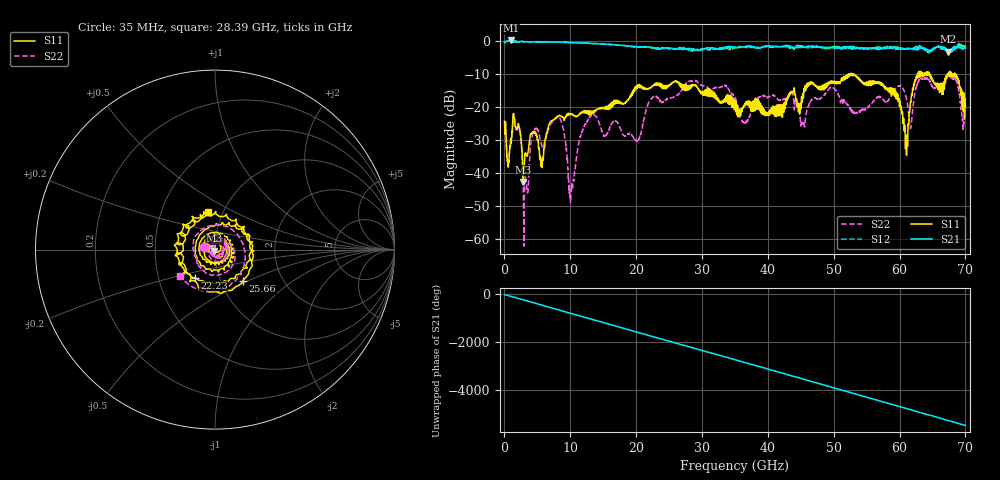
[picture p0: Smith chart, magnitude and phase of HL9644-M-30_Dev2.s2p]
! 7/2/2021 9:55:46 AM
! H:\PRODUCTION_DATA\TEMP_S2P.S2P
! CHANNEL.1
! TR.MEASUREMENT
! CORRECTED.DATA
# GHZ S RI R 50.0
! FREQ.GHZ  S11RE  S11IM  S21RE  S21IM  S12RE  S12IM  S22RE  S22IM
!; PortSelection: Port_12
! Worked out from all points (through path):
!   2000 points, 35 MHz to 70 GHz, reference 50 ohm
!   highest |S21| = 0.04 dB at 1.015 GHz (marker M1); lowest = -3.4 dB at 67.34 GHz (marker M2)
!   group delay of S21, straight-line fit = 217 ps
!   lowest |S11| = -42.8 dB at 2.87 GHz (marker M3), VSWR 1.01, Z = 49.6 - j0.614 ohm
!   |S11| at or under -10 dB: start of sweep to 52.53 GHz; 52.72 GHz to 62.72 GHz (9.998 GHz wide, 17.3 % of centre); 64.56 GHz to 67.42 GHz (2.861 GHz wide, 4.34 % of centre)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
!   |S22| runs from -62.3 to -10.4 dB; largest |S21 - S12| = 0.14
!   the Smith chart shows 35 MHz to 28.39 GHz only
!   S11 on the Smith chart (normalised r, x): 35 MHz: 0.89, +0.03; 22.23 GHz: 0.76, -0.25; 25.66 GHz: 1.27, -0.47; 28.39 GHz: 0.85, +0.37
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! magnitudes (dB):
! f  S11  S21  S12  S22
! 35 MHz  -24.5  -0.6  -0.6  -24.4
! 1.015 GHz  -29.6  0.0  -0.1  -29.6
! 2.205 GHz  -26.3  -0.4  -0.5  -26.7
! 2.87 GHz  -42.8  -0.3  -0.3  -45.0
! 3.29 GHz  -34.1  -0.3  -0.3  -42.1
! 4.515 GHz  -27.5  -0.4  -0.4  -27.2
! 5.705 GHz  -38.5  -0.5  -0.4  -31.9
! 8.12 GHz  -23.1  -0.5  -0.5  -22.9
! 10.12 GHz  -22.2  -0.6  -0.6  -46.3
! 11.72 GHz  -21.7  -0.7  -0.7  -28.4
! 20.16 GHz  -14.1  -1.9  -1.9  -30.3
! 22.23 GHz  -14.3  -2.0  -2.2  -17.8
! 23.38 GHz  -13.5  -2.5  -2.4  -17.3
! 25.66 GHz  -12.6  -2.4  -2.6  -17.2
! 28.39 GHz  -13.4  -2.5  -2.9  -12.3
! 35.03 GHz  -18.2  -2.1  -2.1  -17.3
! 46.69 GHz  -12.7  -1.7  -2.1  -17.9
! 58.34 GHz  -15.5  -2.3  -1.9  -18.2
! 61.04 GHz  -34.5  -2.5  -2.3  -17.6
! 62.76 GHz  -9.9  -2.1  -2.4  -12.6
! 67.34 GHz  -10.7  -3.4  -3.3  -10.4
! 70 GHz  -20.0  -2.2  -2.0  -21.6
